[IBIS Ver]   4.1
[File Name]   sprm687.ibs
[File Rev]   1.0
[Date]   November 15, 2015
[Source]   File originated at Texas Instruments
[Copyright]   (c) 2012, Texas Instruments Inc.
[Component]   f771968xpz
[Manufacturer] Texas Instruments
[Package]
| Variable   Typ   Min   Max
R_pkg   0.251   0.110   0.317
L_pkg   4.95E-09   4.14E-09   5.86E-09
C_pkg   1.23E-12   1.09E-13   1.43E-12
[Pin] signal_name   model_name   R_pin   L_pin   C_pin
1	GPIO28	BCF3385DSHYPBFZ	3.17E-01	5.86E-09	1.16E-12
2	XRSn	BQ0491FS_XRSN_USF 	3.04E-01	5.71E-09	1.33E-12
3	VDDSFL	NC	3.02E-01	5.49E-09	1.32E-12
4	VDD	NC	2.91E-01	5.32E-09	1.29E-12
5	VSS	NC	2.86E-01	5.20E-09	1.24E-12
6	PG5OUTF	ICF33SHYPB_FS_SFII_CUS	3.14E-01	5.53E-09	1.24E-12
7	PG3OUTF	ICF33SHYPB_FS_SFII_CUS	3.07E-01	5.45E-09	1.24E-12
8	B3	ICF33SHYPB_FS_SFII_CUS	2.97E-01	5.16E-09	1.22E-12
9	PG1OUTF	ICF33SHYPB_FS_SFII_CUS	2.88E-01	5.13E-09	1.19E-12
10	A3	ICF33SHYPB_FS_SFII_CUS	2.81E-01	4.95E-09	1.17E-12
11	VDDA	NC	1.62E-01	4.48E-09	1.21E-12
12	VSSA	NC	1.60E-01	4.35E-09	1.20E-12
13	PG5GND	NC	2.66E-01	4.71E-09	1.13E-12
14	PG1GND	NC	2.64E-01	4.62E-09	1.12E-12
15	PG3GND	NC	2.61E-01	4.63E-09	1.13E-12
16	PG5P	NC	2.60E-01	4.63E-09	1.14E-12
17	A14_C4	ICF33SHYPB_USF	2.60E-01	4.67E-09	1.16E-12
18	PG1P	NC	2.62E-01	4.75E-09	1.19E-12
19	A11_B7_C0	ICF33SHYPB_USF	2.66E-01	4.80E-09	1.21E-12
20	PG3P	NC	2.71E-01	4.96E-09	1.24E-12
21	B10_C2	ICF33SHYPB_USF	2.80E-01	5.13E-09	1.27E-12
22	DACOUT2	ICF33SHYPB_USF	2.87E-01	5.26E-09	1.30E-12
23	DACOUT1	ICF33SHYPB_USF	2.98E-01	5.46E-09	1.33E-12
24	VREFHIB	NC	1.82E-01	5.31E-09	1.41E-12
25	VREFHIA	NC	1.86E-01	5.39E-09	1.20E-12
26	VREFLOB	NC	1.88E-01	5.45E-09	1.20E-12
27	VREFLOA	NC	1.85E-01	5.32E-09	1.43E-12
28	A15_C5	ICF33SHYPB_USF	1.79E-01	5.19E-09	1.41E-12
29	A12_B9_C1	ICF33SHYPB_USF	2.89E-01	5.35E-09	1.31E-12
30	PG2P	NC	2.80E-01	5.09E-09	1.28E-12
31	B11_C3	ICF33SHYPB_USF	1.64E-01	4.56E-09	1.31E-12
32	PG4GND	NC	1.25E-01	4.31E-09	1.33E-12
33	VSSA	NC	1.59E-01	4.45E-09	1.26E-12
34	VDDA	NC	1.56E-01	4.35E-09	1.23E-12
35	A5	ICF33SHYPB_FS_SFII_CUS	2.61E-01	4.66E-09	1.14E-12
36	PG2OUTF	ICF33SHYPB_FS_SFII_CUS	2.58E-01	4.56E-09	1.12E-12
37	PG6OUTF	ICF33SHYPB_FS_SFII_CUS	2.59E-01	4.66E-09	1.10E-12
38	A9	ICF33SHYPB_FS_SFII_CUS	2.57E-01	4.58E-09	1.11E-12
39	PG4OUTF	ICF33SHYPB_FS_SFII_CUS	2.60E-01	4.60E-09	1.11E-12
40	PG7OUTF	ICF33SHYPB_FS_SFII_CUS	2.61E-01	4.59E-09	1.13E-12
41	B0	ICF33SHYPB_FS_SFII_CUS	2.65E-01	4.75E-09	1.14E-12
42	PG7GND	NC	2.70E-01	4.81E-09	1.17E-12
43	PG7P	NC	2.76E-01	4.96E-09	1.20E-12
44	B12_C14	ICF33SHYPB_USF	2.85E-01	5.22E-09	1.21E-12
45	VSS	NC	2.83E-01	5.12E-09	1.24E-12
46	VDD	NC	2.88E-01	5.17E-09	1.28E-12
47	VDDSFL	NC	1.37E-01	4.82E-09	1.37E-12
48	FLT2	NC	2.92E-01	5.37E-09	1.31E-12
49	FLT1	NC	3.01E-01	5.61E-09	1.33E-12
50	GPIO13	BCPF335585DSHYPBFZ	3.09E-01	5.79E-09	1.15E-12
51	GPIO12	BCF3385DSHYPBFZ	3.07E-01	5.65E-09	1.15E-12
52	GPIO11	BCPF335585DSHYPBFZ	2.90E-01	5.43E-09	1.35E-12
53	GPIO33	BCPF335585DSHYPBFZ	2.81E-01	5.23E-09	1.32E-12
54	GPIO16	BT3308BT5FSHYPB_SFII	2.69E-01	5.02E-09	1.27E-12
55	GPIO17	BT3308BT5FSHYPB_SFII	2.65E-01	4.91E-09	1.24E-12
56	GPIO24	BT3308BT5FSHYPB_SFII	2.62E-01	4.79E-09	1.22E-12
57	GPIO25	BT3308BT5FSHYPB_SFII	2.60E-01	4.74E-09	1.19E-12
58	GPIO26	BT3308BT5FSHYPB_SFII	2.59E-01	4.76E-09	1.16E-12
59	GPIO27	BT3308BT5FSHYPB_SFII	2.59E-01	4.70E-09	1.13E-12
60	TCK	BCF3355DSHYPBFZ_TMS_USF 	2.58E-01	4.63E-09	1.13E-12
61	GPIO37_TDO	BT3308BT5FSHYPB_SFII	2.59E-01	4.72E-09	1.12E-12
62	TMS	BCF3355DSHYPBFZ_TMS_USF 	2.61E-01	4.61E-09	1.11E-12
63	GPIO35_TDI	BT3308BT5FSHYPB_SFII	2.64E-01	4.63E-09	1.10E-12
64	GPIO32	BCF3385DSHYPBFZ_USF	2.61E-01	4.63E-09	1.09E-12
65	GPIO56	BCF3385DSHYPBFZ_USF	2.61E-01	4.67E-09	1.11E-12
66	GPIO57	BCF3385DSHYPBFZ_USF	2.64E-01	4.66E-09	1.14E-12
67	GPIO58	BCF3385DSHYPBFZ_USF	2.69E-01	4.79E-09	1.16E-12
68	X2_GPIO18	BCF3385DSHYPBFZ_USF	1.61E-01	4.41E-09	1.24E-12
69	X1_GPIO19	BCF3385DSHYPBFZ_USF	1.64E-01	4.51E-09	1.30E-12
70	VDDSFL	NC	1.27E-01	4.43E-09	1.36E-12
71	VDD	NC	1.10E-01	4.34E-09	1.42E-12
72	VSS	NC	2.82E-01	5.18E-09	1.29E-12
73	VREGENZ	IQ0440FS_VREGENZ_USF	2.82E-01	5.26E-09	1.29E-12
74	GPIO8	BCF3385DSHYPBFZ	2.92E-01	5.58E-09	1.33E-12
75	GPIO4	BCPF335585DSHYPBFZ	3.08E-01	5.69E-09	1.15E-12
76	GPIO3	BCPF335585DSHYPBFZ	3.10E-01	5.82E-09	1.15E-12
77	GPIO2	BCPF335585DSHYPBFZ	3.00E-01	5.60E-09	1.35E-12
78	GPIO1	BCPF335585DSHYPBFZ	2.88E-01	5.31E-09	1.33E-12
79	GPIO0	BCPF335585DSHYPBFZ	2.79E-01	5.11E-09	1.28E-12
80	VDDSW33	NC	1.31E-01	4.60E-09	1.35E-12
81	VOUTSW33_GPIO23	BCF3335DSHYPBFZ	1.29E-01	4.48E-09	1.36E-12
82	VSS_DCDC	NC	1.26E-01	4.40E-09	1.30E-12
83	VFB_DCDC_GPIO22	BCF3385DSHYPBFZ	2.74E-01	4.84E-09	1.16E-12
84	GPIO7	BCF3385DSHYPBFZ_USF	2.83E-01	4.94E-09	1.16E-12
85	GPIO40	BT3308BT5FSHYPB_SFII	2.75E-01	4.86E-09	1.15E-12
86	VSS	NC	2.76E-01	4.78E-09	1.13E-12
87	VDD	NC	1.22E-01	4.14E-09	1.21E-12
88	VDDSFL	NC	1.59E-01	4.25E-09	1.17E-12
89	GPIO5	BCPF335585DSHYPBFZ	2.79E-01	4.80E-09	1.12E-12
90	GPIO9	BCF3385DSHYPBFZ	2.71E-01	4.71E-09	1.15E-12
91	GPIO39	BCF3385DSHYPBFZ_USF	2.63E-01	4.62E-09	1.15E-12
92	GPIO59	BCF3385DSHYPBFZ_USF	2.59E-01	4.60E-09	1.16E-12
93	GPIO10	BCF3385DSHYPBFZ_USF	2.58E-01	4.69E-09	1.18E-12
94	GPIO34	BCF3385DSHYPBFZ_USF	2.57E-01	4.69E-09	1.20E-12
95	GPIO15	BCF3385DSHYPBFZ_USF	2.59E-01	4.79E-09	1.22E-12
96	GPIO14	BCF3385DSHYPBFZ_USF	2.61E-01	4.85E-09	1.24E-12
97	GPIO6	BCF3385DSHYPBFZ_USF	2.65E-01	4.96E-09	1.27E-12
98	GPIO30	BCF3385DSHYPBFZ	2.81E-01	5.32E-09	1.33E-12
99	GPIO31	BCF3385DSHYPBFZ	2.98E-01	5.55E-09	1.38E-12
100	GPIO29	BCPF335585DSHYPBFZ	3.16E-01	5.79E-09	1.18E-12
| End of package information
|   Component IQ0440FS_VREGENZ_USF
[Component]   IQ0440FS_VREGENZ_USF
[Manufacturer]   Texas Instruments
[Package]
|  variable   typ   min   max
R_pkg   0   0   0
L_pkg   0   0   0
C_pkg   0   0   0
[Pin]   signal_name   model_name   R_pin   L_pin   C_pin
VSS   VSS   GND
VDDS   VDDS   POWER
PAD   PAD   IQ0440FS_VREGENZ_USF
[Model Selector] IQ0440FS_VREGENZ_USF
VREGENZ_WK_PD_ON_3P3  Cell operated at 3.3(nom)
|VREGENZ_WK_PD_ON_3P3; WEAK_PULLDOWN_ON
VREGENZ_WK_PD_OFF_3P3  Cell operated at 3.3(nom)
|   Component ICF33SHYPB_USF
[Component]   ICF33SHYPB_USF
[Manufacturer]   Texas Instruments
[Package]
|  variable   typ   min   max
R_pkg   0   0   0
L_pkg   0   0   0
C_pkg   0   0   0
[Pin]   signal_name   model_name   R_pin   L_pin   C_pin
VSS   VSS   GND
VDDS   VDDS   POWER
PAD   PAD   ICF33SHYPB_USF
[Model Selector] ICF33SHYPB_USF
ICF_WK_PUPD_OFF_3P3  Cell operated at 3.3(nom)
|ICF_WK_PUPD_OFF_3P3; WEAK_PULL_OFF
ICF_WK_PU_ON_3P3  Cell operated at 3.3(nom)
|ICF_WK_PU_ON_3P3; WEAK_PULLUP_ON
ICF_WK_PD_ON_3P3  Cell operated at 3.3(nom)
|   Component ICF33SHYPB_FS_SFII_CUS
[Component]   ICF33SHYPB_FS_SFII_CUS
[Manufacturer]   Texas Instruments
[Package]
|  variable   typ   min   max
R_pkg   0   0   0
L_pkg   0   0   0
C_pkg   0   0   0
[Pin]   signal_name   model_name   R_pin   L_pin   C_pin
VSS   VSS   GND
VDDS   VDDS   POWER
PAD   PAD   ICF33SHYPB_FS_SFII_CUS
[Model Selector] ICF33SHYPB_FS_SFII_CUS
CUS_WK_PUPD_OFF_3P3  Cell operated at 3.3(nom)
|CUS_WK_PUPD_OFF_3P3; WEAK_PULL_OFF
CUS_WK_PU_ON_3P3  Cell operated at 3.3(nom)
|CUS_WK_PU_ON_3P3; WEAK_PULLUP_ON
CUS_WK_PD_ON_3P3  Cell operated at 3.3(nom)
|   Component BT3308BT5FSHYPB_SFII
[Component]   BT3308BT5FSHYPB_SFII
[Manufacturer]   Texas Instruments
[Package]
|  variable   typ   min   max
R_pkg   0   0   0
L_pkg   0   0   0
C_pkg   0   0   0
[Pin]   signal_name   model_name   R_pin   L_pin   C_pin
VSS   VSS   GND
VDDS   VDDS   POWER
PAD   PAD   BT3308BT5FSHYPB_SFII
[Model Selector] BT3308BT5FSHYPB_SFII
BT_OPEN_DRAIN_6MA_3P3  Cell operated at 3.3(nom)
|BT_OPEN_DRAIN_6MA_3P3
BT_WEAK_PD_ON_3P3  Cell operated at 3.3(nom)
|BT_WEAK_PD_ON_3P3
BT_OPEN_DRAIN_3MA_3P3  Cell operated at 3.3(nom)
|BT_OPEN_DRAIN_3MA_3P3
BT_DRIVER_MODE_6MA_3P3  Cell operated at 3.3(nom)
|BT_DRIVER_MODE_6MA_3P3
BT_DRIVER_MODE_3MA_3P3  Cell operated at 3.3(nom)
|BT_DRIVER_MODE_3MA_3P3
BT_WEAK_PU_ON_3P3  Cell operated at 3.3(nom)
|   Component BQ0491FS_XRSN_USF
[Component]   BQ0491FS_XRSN_USF
[Manufacturer]   Texas Instruments
[Package]
|  variable   typ   min   max
R_pkg   0   0   0
L_pkg   0   0   0
C_pkg   0   0   0
[Pin]   signal_name   model_name   R_pin   L_pin   C_pin
VSS   VSS   GND
VDDS   VDDS   POWER
PAD   PAD   BQ0491FS_XRSN_USF
[Model Selector] BQ0491FS_XRSN_USF
XRSN_WK_PU_ON_3P3  Cell operated at 3.3(nom)
|XRSN_WK_PU_ON_3P3; WEAK_PULLUP_ON
XRSN_OPEN_DRAIN  Cell operated at 3.3(nom)
|   Component BCPF335585DSHYPBFZ
[Component]   BCPF335585DSHYPBFZ
[Manufacturer]   Texas Instruments
[Package]
|  variable   typ   min   max
R_pkg   0   0   0
L_pkg   0   0   0
C_pkg   0   0   0
[Pin]   signal_name   model_name   R_pin   L_pin   C_pin
VSS   VSS   GND
VDDS   VDDS   POWER
PAD   PAD   BCPF335585DSHYPBFZ
[Model Selector] BCPF335585DSHYPBFZ
BCPF_WK_PU_ON_3P3  Cell operated at 3.3(nom)
|BCPF_WK_PU_ON_3P3; WEAK_PULLUP_ON
BCPF_DRIVER_4MA_3P3  Cell operated at 3.3(nom)
|BCPF_DRIVER_4MA_3P3
BCPF_DRIVER_2MA_3P3  Cell operated at 3.3(nom)
|BCPF_DRIVER_2MA_3P3
BCPF_WK_PD_ON_3P3  Cell operated at 3.3(nom)
|   Component BCF3385DSHYPBFZ_USF
[Component]   BCF3385DSHYPBFZ_USF
[Manufacturer]   Texas Instruments
[Package]
|  variable   typ   min   max
R_pkg   0   0   0
L_pkg   0   0   0
C_pkg   0   0   0
[Pin]   signal_name   model_name   R_pin   L_pin   C_pin
VSS   VSS   GND
VDDS   VDDS   POWER
PAD   PAD   BCF3385DSHYPBFZ_USF
[Model Selector] BCF3385DSHYPBFZ_USF
BCF3385DUSF_WK_PU  Cell operated at 3.3(nom)
| BCF3385DUSF_WK_PU; WEAK_PULLUP_ON
BCF3385DUSF_DRIVER_3P3  Cell operated at 3.3(nom)
|BCF3385DUSF_DRIVER_3P3
BCF3385DUSF_WK_PD  Cell operated at 3.3(nom)
|   Component BCF3385DSHYPBFZ
[Component]   BCF3385DSHYPBFZ
[Manufacturer]   Texas Instruments
[Package]
|  variable   typ   min   max
R_pkg   0   0   0
L_pkg   0   0   0
C_pkg   0   0   0
[Pin]   signal_name   model_name   R_pin   L_pin   C_pin
VSS   VSS   GND
VDDS   VDDS   POWER
PAD   PAD   BCF3385DSHYPBFZ
[Model Selector] BCF3385DSHYPBFZ
BCF3385D_WK_PU_3P3  Cell operated at 3.3(nom)
|BCF3385D_WK_PU_3P3; WEAK_PULLUP_ON
BCF3385D_DRIVER_3P3  Cell operated at 3.3(nom)
|BCF3385D_DRIVER_3P3
BCF3385D_WK_PD_3P3  Cell operated at 3.3(nom)
|   Component BCF3355DSHYPBFZ_TMS_USF
[Component]   BCF3355DSHYPBFZ_TMS_USF
[Manufacturer]   Texas Instruments
[Package]
|  variable   typ   min   max
R_pkg   0   0   0
L_pkg   0   0   0
C_pkg   0   0   0
[Pin]   signal_name   model_name   R_pin   L_pin   C_pin
VSS   VSS   GND
VDDS   VDDS   POWER
PAD   PAD   BCF3355DSHYPBFZ_TMS_USF
[Model Selector] BCF3355DSHYPBFZ_TMS_USF
TMS_WK_PU_ON_3P3  Cell operated at 3.3(nom)
|TMS_WK_PU_ON_3P3; WEAK_PULLUP_ON
TMS_DRIVER_3P3  Cell operated at 3.3(nom)
|TMS_DRIVER_3P3
TMS_WK_PD_ON_3P3  Cell operated at 3.3(nom)
|   Component BCF3335DSHYPBFZ
[Component]   BCF3335DSHYPBFZ
[Manufacturer]   Texas Instruments
[Package]
|  variable   typ   min   max
R_pkg   0   0   0
L_pkg   0   0   0
C_pkg   0   0   0
[Pin]   signal_name   model_name   R_pin   L_pin   C_pin
VSS   VSS   GND
VDDS   VDDS   POWER
PAD   PAD   BCF3335DSHYPBFZ
[Model Selector] BCF3335DSHYPBFZ
BCF3335D_WK_PU_3P3  Cell operated at 3.3(nom)
|BCF3335D_WK_PU_3P3; WEAK_PULLUP_ON
BCF3335D_DRIVER_3P3  Cell operated at 3.3(nom)
|BCF3335D_DRIVER_3P3
BCF3335D_WK_PD_3P3  Cell operated at 3.3(nom)
| Models and submodels in the file (32): VREGENZ_WK_PD_ON_3P3 (Input), VREGENZ_WK_PD_OFF_3P3 (Input), ICF_WK_PUPD_OFF_3P3 (Input), ICF_WK_PU_ON_3P3 (Input), ICF_WK_PD_ON_3P3 (Input), CUS_WK_PUPD_OFF_3P3 (Input), CUS_WK_PU_ON_3P3 (Input), CUS_WK_PD_ON_3P3 (Input), BT_OPEN_DRAIN_6MA_3P3 (I/O_open_drain), BT_WEAK_PD_ON_3P3 (Input), BT_OPEN_DRAIN_3MA_3P3 (I/O_open_drain), BT_DRIVER_MODE_6MA_3P3 (I/O), BT_DRIVER_MODE_3MA_3P3 (I/O), BT_WEAK_PU_ON_3P3 (Input), XRSN_WK_PU_ON_3P3 (Input), XRSN_OPEN_DRAIN (I/O_open_drain), BCPF_WK_PU_ON_3P3 (Input), BCPF_DRIVER_4MA_3P3 (I/O), BCPF_DRIVER_2MA_3P3 (I/O), BCPF_WK_PD_ON_3P3 (Input), BCF3385DUSF_WK_PU (Input), BCF3385DUSF_DRIVER_3P3 (I/O), BCF3385DUSF_WK_PD (Input), BCF3385D_WK_PU_3P3 (Input), BCF3385D_DRIVER_3P3 (I/O), BCF3385D_WK_PD_3P3 (Input), TMS_WK_PU_ON_3P3 (Input), TMS_DRIVER_3P3 (I/O), TMS_WK_PD_ON_3P3 (Input), BCF3335D_WK_PU_3P3 (Input), BCF3335D_DRIVER_3P3 (I/O), BCF3335D_WK_PD_3P3 (Input)
